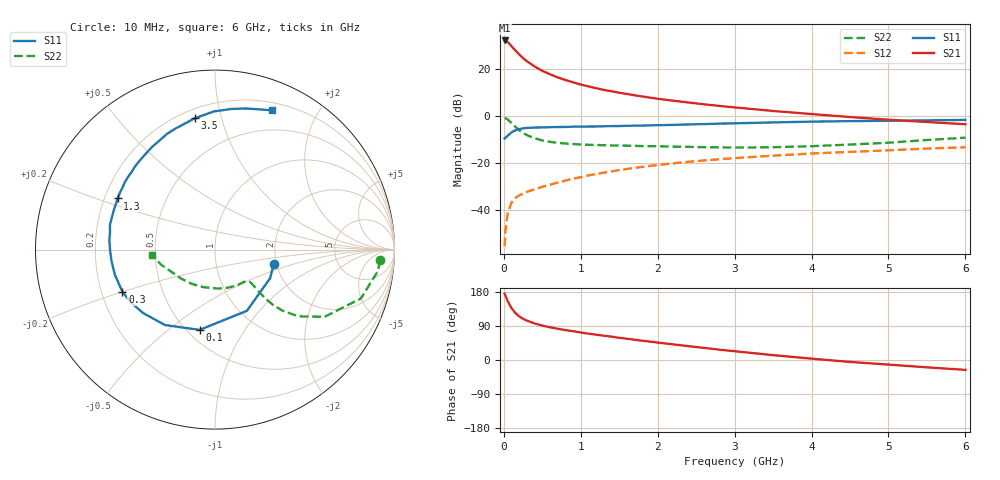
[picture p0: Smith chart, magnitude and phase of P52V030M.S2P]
! SIEMENS Small Signal Semiconductors
! BFP183
! Si NPN RF Bipolar Junction Transistor in SOT143
! VCE = 2 V  IC = 30 mA
! Common Emitter S-Parameters:  March  1996
# GHz  S  MA  R  50
!  f  S11  S21  S12  S22
! GHz  MAG  ANG  MAG  ANG  MAG  ANG  MAG  ANG
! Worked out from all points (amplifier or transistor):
!   36 points, 10 MHz to 6 GHz, reference 50 ohm
!   highest |S21| = 32.4 dB at 10 MHz (marker M1)
!   |S21| within 3 dB of that: start of sweep to 115.5 MHz
!   unconditionally stable (mu >= 1): 507.3 MHz to 5.966 GHz
!   at 250 MHz: K = 0.67, MSG = 28.9 dB, |S12| = -33.0 dB
!   at 1.4 GHz: K = 1.25, MAG = 14.1 dB, |S12| = -23.5 dB
!   at 6 GHz: K = 1.00, MSG = 4.9 dB, |S12| = -13.2 dB
!   S11 on the Smith chart (normalised r, x): 10 MHz: 1.93, -0.35; 100 MHz: 0.57, -0.65; 300 MHz: 0.29, -0.20; 1.3 GHz: 0.25, +0.23; 3.5 GHz: 0.25, +0.83; 6 GHz: 0.28, +1.45
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0.01  0.3368 -13.8  41.48 174.9  0.0017 76.9  0.9233 -3.7
0.02  0.346 -27.4  41.21 170.0  0.0036 83.1  0.9141 -7.7
0.05  0.3846 -62.5  38.51 155.3  0.0086 71.4  0.8574 -18.5
0.1  0.4553 -100.9  31.35 136.8  0.0146 58.6  0.7165 -31.5
0.15  0.5042 -123.5  25.4 124.0  0.0182 53.7  0.5946 -38.7
0.2  0.5344 -138.6  20.84 115.1  0.0206 50.6  0.5056 -42.2
0.25  0.5532 -147.8  17.42 108.6  0.0225 50.0  0.4415 -43.7
0.3  0.5668 -155.5  14.96 103.9  0.0246 49.7  0.3961 -44.1
0.4  0.5753 -165.9  11.56 96.4  0.0277 51.3  0.34 -43.9
0.5  0.5802 -173.8  9.307 90.9  0.0315 52.2  0.3062 -43.3
0.6  0.5851 180.0  7.876 86.3  0.0348 54.8  0.2852 -42.9
0.7  0.591 174.8  6.749 82.5  0.0386 56.2  0.2715 -42.7
0.8  0.5932 170.5  5.955 78.9  0.0426 56.5  0.263 -43.0
1.1  0.6055 158.5  4.345 69.5  0.055 57.8  0.2468 -45.6
1.3  0.6131 152.3  3.664 64.1  0.0628 57.1  0.242 -48.4
1.7  0.6321 139.7  2.808 53.5  0.0793 54.8  0.2347 -55.8
2.2  0.6571 126.6  2.156 41.2  0.0994 51.3  0.2257 -67.4
2.8  0.6984 112.4  1.666 27.3  0.1213 45.7  0.2181 -84.4
3.5  0.7407 98.6  1.299 12.8  0.145 39.3  0.2189 -107.2
4.5  0.7892 83.3  0.966 -5.1  0.1742 29.8  0.2498 -140.3
5.5  0.8193 72.5  0.756 -19.4  0.2054 21.4  0.3124 -164.5
6  0.8381 67.8  0.677 -26.0  0.2184 16.6  0.35 -174.9
